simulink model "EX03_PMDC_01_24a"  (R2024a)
settings: Solver=ode45  StartTime=0.0  StopTime=0.2  MaxStep=1e-5  RelTol=1e-3  EnableMultiTasking=on
libraries: spsControlledVoltageSourceLib x1, spsDCMachineLib x1, spspowerguiLib x1

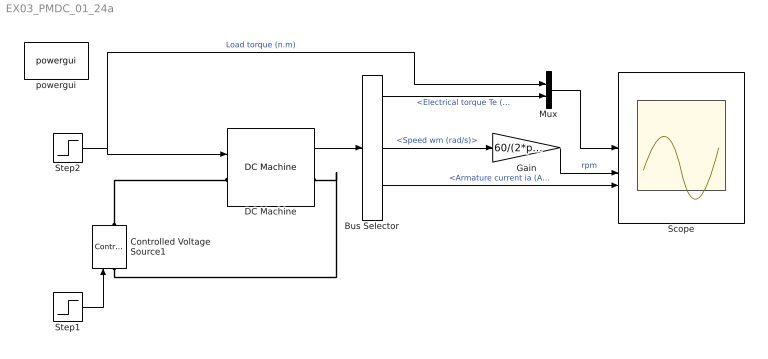
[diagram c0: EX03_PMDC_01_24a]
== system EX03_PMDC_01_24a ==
  Bus Selector : BusSelector  OutputSignals=Electrical torque Te (n m),Speed wm (rad/s),Armature current ia (A)
  Controlled Voltage Source1 : spsControlledVoltageSourceLib/Controlled Voltage Source  Initialize=on  Source_Type=AC  Amplitude=0  Phase=0  Frequency=0  Measurements=Voltage
  DC Machine : spsDCMachineLib/DC Machine  PresetModel=No  MechanicalLoad=Torque TL  FieldType=Permanent magnet  ShowDetailedParameters=on  MeasurementBus=off  RLa=[0.26 1.7e-3]  RLf="[ 240  120]"  Laf=1.8  MachineConstant=Back-emf constant (V/rpm)  Ke=0.04415  Kt=1.8  J=0.00252  Bm=0  Tf=0  w0=0  Ifinit=1  TsPowergui=0  TsBlock=-1
  Gain : Gain  Gain=60/(2*pi)
  Mux : Mux  Inputs=2
  Scope : Scope  NumInputPorts=3
  Step1 : Step  Time=0  After=139  SampleTime=0
  Step2 : Step  Time=0.1  After=9.8039  SampleTime=0
  powergui : spspowerguiLib/powergui  Priority=1  SimulationMode=Continuous  SampleTime=50e-6  frequency=60  Iterations=50  frequencyindice=0  Pbase=100e6  ErrMax=1e-4  UnitsV=kV  UnitsW=MW  buscounter=0  FunctionMessages=off  echomessages=off  EnableUseOfTLC=off  CurrentSourceSwitches=off  DisableSnubberDevices=on  DisableRonSwitches=on  DisableVfSwitches=on  DisplayEquations=off  AutomaticDiscreteSolvers=off  SolverType=Tustin  Interpol=off  ExternalGateDelay=off  methode=off  Ts=0  x0status=blocks  SPID=on  SwTol=0  HookPort=off  NonlinearTolerance=1e-4  nMaxIteration=100  ContinueOnMaxIteration=off  RestoreLinks=warning  ResistiveCurrentMeasurement=off  Frange=[0:2:500]  Ylog=off  Xlog=on  ShowGrid=off  save=off  variable=ZData  structure=0  ZoomFFT=off  StartTime=0.0  cycles=1  DisplayStyle=1  fundamental=60  FreqAxis=off  MaxFrequency=1000  frequencyindicesteady=1  RmsSteady=1  display=off
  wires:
  Step1/1 -> Controlled Voltage Source1/1
  DC Machine/1 -> Bus Selector/1
  Bus Selector/2 -> Gain/1  "<Speed wm (rad/s)>"
  Bus Selector/3 -> Scope/3  "<Armature current ia (A)>"
  Gain/1 -> Scope/2  "rpm"
  Step2/1 -> DC Machine/1, Mux/1  "Load torque (n.m)"
  Mux/1 -> Scope/1
  Bus Selector/1 -> Mux/2  "<Electrical torque Te (n m)>"
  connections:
  Controlled Voltage Source1/LConn1 -- DC Machine/RConn1
  Controlled Voltage Source1/RConn1 -- DC Machine/LConn1
